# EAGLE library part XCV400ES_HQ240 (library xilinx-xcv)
xcv400es_hq240 edit this description Auto generated by make-symbol-device-package-bsdl.ulp Rev. 26 Source: xcv400es_hq240.bsd
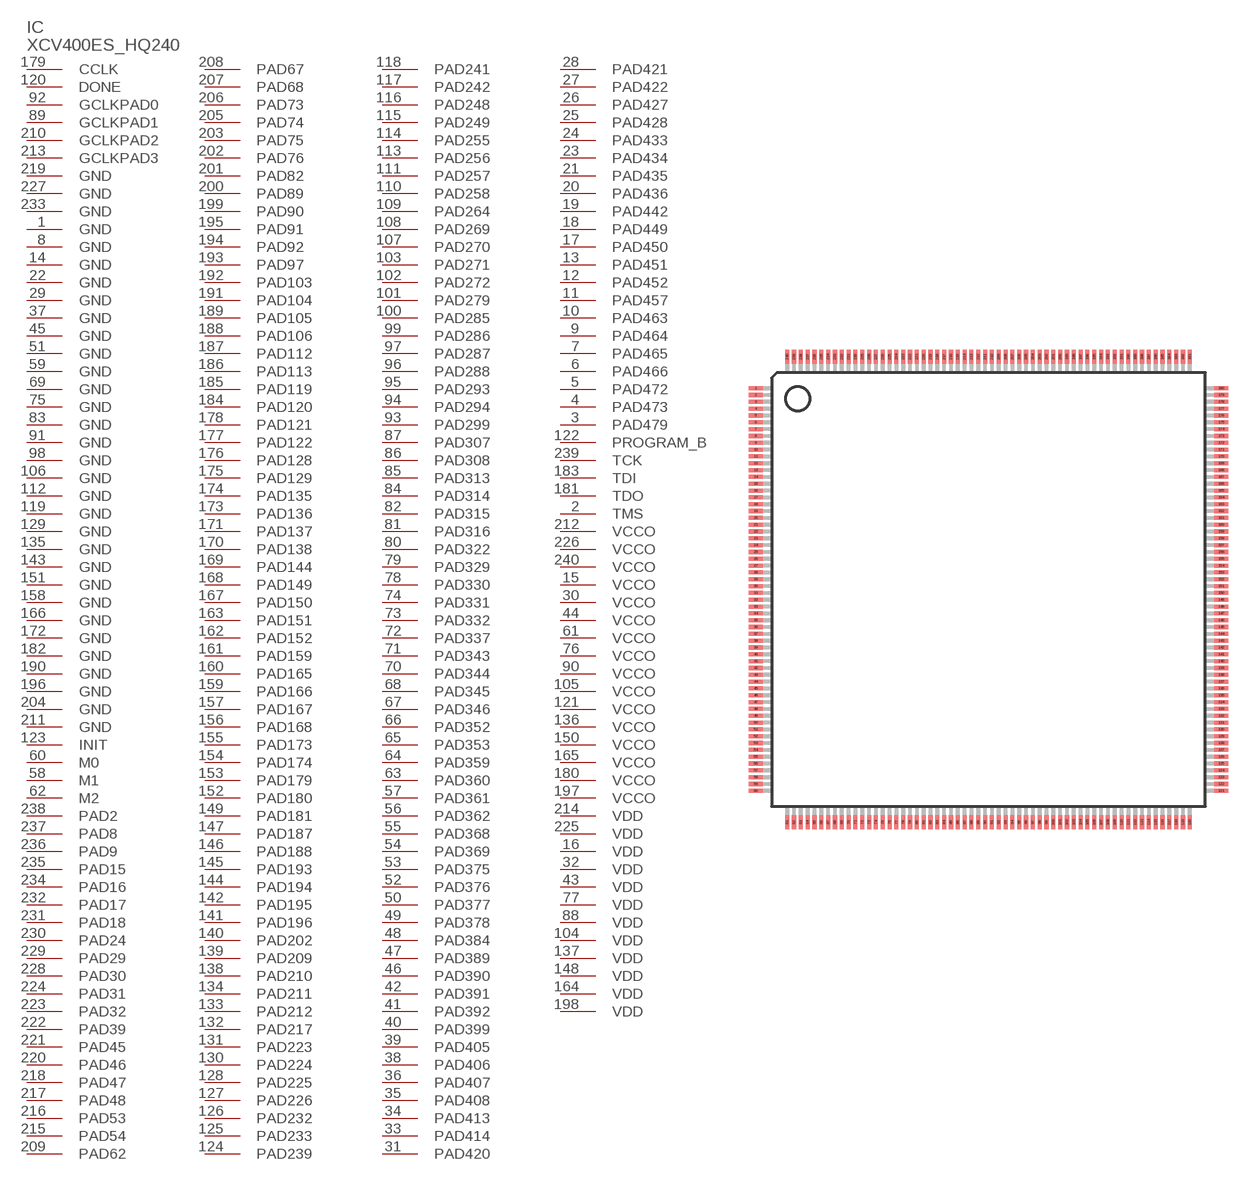
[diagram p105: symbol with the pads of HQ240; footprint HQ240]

Designator prefix IC

## XCV400ES_HQ240 (OC_FARNELL: unknown; OC_NEWARK: unknown)  [HQ240]
1  GND  pwr
2  TMS  in
3  PAD479
4  PAD473
5  PAD472
6  PAD466
7  PAD465
8  GND  pwr
9  PAD464
10  PAD463
11  PAD457
12  PAD452
13  PAD451
14  GND  pwr
15  VCCO  pwr
16  VDD  pwr
17  PAD450
18  PAD449
19  PAD442
20  PAD436
21  PAD435
22  GND  pwr
23  PAD434
24  PAD433
25  PAD428
26  PAD427
27  PAD422
28  PAD421
29  GND  pwr
30  VCCO  pwr
31  PAD420
32  VDD  pwr
33  PAD414
34  PAD413
35  PAD408
36  PAD407
37  GND  pwr
38  PAD406
39  PAD405
40  PAD399
41  PAD392
42  PAD391
43  VDD  pwr
44  VCCO  pwr
45  GND  pwr
46  PAD390
47  PAD389
48  PAD384
49  PAD378
50  PAD377
51  GND  pwr
52  PAD376
53  PAD375
54  PAD369
55  PAD368
56  PAD362
57  PAD361
58  M1  in
59  GND  pwr
60  M0  in
61  VCCO  pwr
62  M2  in
63  PAD360
64  PAD359
65  PAD353
66  PAD352
67  PAD346
68  PAD345
69  GND  pwr
70  PAD344
71  PAD343
72  PAD337
73  PAD332
74  PAD331
75  GND  pwr
76  VCCO  pwr
77  VDD  pwr
78  PAD330
79  PAD329
80  PAD322
81  PAD316
82  PAD315
83  GND  pwr
84  PAD314
85  PAD313
86  PAD308
87  PAD307
88  VDD  pwr
89  GCLKPAD1  in
90  VCCO  pwr
91  GND  pwr
92  GCLKPAD0  in
93  PAD299
94  PAD294
95  PAD293
96  PAD288
97  PAD287
98  GND  pwr
99  PAD286
100  PAD285
101  PAD279
102  PAD272
103  PAD271
104  VDD  pwr
105  VCCO  pwr
106  GND  pwr
107  PAD270
108  PAD269
109  PAD264
110  PAD258
111  PAD257
112  GND  pwr
113  PAD256
114  PAD255
115  PAD249
116  PAD248
117  PAD242
118  PAD241
119  GND  pwr
120  DONE
121  VCCO  pwr
122  PROGRAM_B  in
123  INIT
124  PAD239
125  PAD233
126  PAD232
127  PAD226
128  PAD225
129  GND  pwr
130  PAD224
131  PAD223
132  PAD217
133  PAD212
134  PAD211
135  GND  pwr
136  VCCO  pwr
137  VDD  pwr
138  PAD210
139  PAD209
140  PAD202
141  PAD196
142  PAD195
143  GND  pwr
144  PAD194
145  PAD193
146  PAD188
147  PAD187
148  VDD  pwr
149  PAD181
150  VCCO  pwr
151  GND  pwr
152  PAD180
153  PAD179
154  PAD174
155  PAD173
156  PAD168
157  PAD167
158  GND  pwr
159  PAD166
160  PAD165
161  PAD159
162  PAD152
163  PAD151
164  VDD  pwr
165  VCCO  pwr
166  GND  pwr
167  PAD150
168  PAD149
169  PAD144
170  PAD138
171  PAD137
172  GND  pwr
173  PAD136
174  PAD135
175  PAD129
176  PAD128
177  PAD122
178  PAD121
179  CCLK
180  VCCO  pwr
181  TDO  out
182  GND  pwr
183  TDI  in
184  PAD120
185  PAD119
186  PAD113
187  PAD112
188  PAD106
189  PAD105
190  GND  pwr
191  PAD104
192  PAD103
193  PAD97
194  PAD92
195  PAD91
196  GND  pwr
197  VCCO  pwr
198  VDD  pwr
199  PAD90
200  PAD89
201  PAD82
202  PAD76
203  PAD75
204  GND  pwr
205  PAD74
206  PAD73
207  PAD68
208  PAD67
209  PAD62
210  GCLKPAD2  in
211  GND  pwr
212  VCCO  pwr
213  GCLKPAD3  in
214  VDD  pwr
215  PAD54
216  PAD53
217  PAD48
218  PAD47
219  GND  pwr
220  PAD46
221  PAD45
222  PAD39
223  PAD32
224  PAD31
225  VDD  pwr
226  VCCO  pwr
227  GND  pwr
228  PAD30
229  PAD29
230  PAD24
231  PAD18
232  PAD17
233  GND  pwr
234  PAD16
235  PAD15
236  PAD9
237  PAD8
238  PAD2
239  TCK  in
240  VCCO  pwr

## Footprint HQ240 (pad centres in mm)
HQ240 Auto generated by make-symbol-device-package-bsdl.ulp Rev. 26
smd 1 x 0.3: 1 -17.05,14.75; 2 -17.05,14.25; 3 -17.05,13.75; 4 -17.05,13.25; 5 -17.05,12.75; 6 -17.05,12.25; 7 -17.05,11.75; 8 -17.05,11.25; 9 -17.05,10.75; 10 -17.05,10.25; 11 -17.05,9.75; 12 -17.05,9.25; 13 -17.05,8.75; 14 -17.05,8.25; 15 -17.05,7.75; 16 -17.05,7.25; 17 -17.05,6.75; 18 -17.05,6.25; 19 -17.05,5.75; 20 -17.05,5.25; 21 -17.05,4.75; 22 -17.05,4.25; 23 -17.05,3.75; 24 -17.05,3.25; 25 -17.05,2.75; 26 -17.05,2.25; 27 -17.05,1.75; 28 -17.05,1.25; 29 -17.05,0.75; 30 -17.05,0.25; 31 -17.05,-0.25; 32 -17.05,-0.75; 33 -17.05,-1.25; 34 -17.05,-1.75; 35 -17.05,-2.25; 36 -17.05,-2.75; 37 -17.05,-3.25; 38 -17.05,-3.75; 39 -17.05,-4.25; 40 -17.05,-4.75; 41 -17.05,-5.25; 42 -17.05,-5.75; 43 -17.05,-6.25; 44 -17.05,-6.75; 45 -17.05,-7.25; 46 -17.05,-7.75; 47 -17.05,-8.25; 48 -17.05,-8.75; 49 -17.05,-9.25; 50 -17.05,-9.75; 51 -17.05,-10.25; 52 -17.05,-10.75; 53 -17.05,-11.25; 54 -17.05,-11.75; 55 -17.05,-12.25; 56 -17.05,-12.75; 57 -17.05,-13.25; 58 -17.05,-13.75; 59 -17.05,-14.25; 60 -17.05,-14.75; 121 17.05,-14.75; 122 17.05,-14.25; 123 17.05,-13.75; 124 17.05,-13.25; 125 17.05,-12.75; 126 17.05,-12.25; 127 17.05,-11.75; 128 17.05,-11.25; 129 17.05,-10.75; 130 17.05,-10.25; 131 17.05,-9.75; 132 17.05,-9.25; 133 17.05,-8.75; 134 17.05,-8.25; 135 17.05,-7.75; 136 17.05,-7.25; 137 17.05,-6.75; 138 17.05,-6.25; 139 17.05,-5.75; 140 17.05,-5.25; 141 17.05,-4.75; 142 17.05,-4.25; 143 17.05,-3.75; 144 17.05,-3.25; 145 17.05,-2.75; 146 17.05,-2.25; 147 17.05,-1.75; 148 17.05,-1.25; 149 17.05,-0.75; 150 17.05,-0.25; 151 17.05,0.25; 152 17.05,0.75; 153 17.05,1.25; 154 17.05,1.75; 155 17.05,2.25; 156 17.05,2.75; 157 17.05,3.25; 158 17.05,3.75; 159 17.05,4.25; 160 17.05,4.75; 161 17.05,5.25; 162 17.05,5.75; 163 17.05,6.25; 164 17.05,6.75; 165 17.05,7.25; 166 17.05,7.75; 167 17.05,8.25; 168 17.05,8.75; 169 17.05,9.25; 170 17.05,9.75; 171 17.05,10.25; 172 17.05,10.75; 173 17.05,11.25; 174 17.05,11.75; 175 17.05,12.25; 176 17.05,12.75; 177 17.05,13.25; 178 17.05,13.75; 179 17.05,14.25; 180 17.05,14.75
smd 0.3 x 1: 61 -14.75,-17.05; 62 -14.25,-17.05; 63 -13.75,-17.05; 64 -13.25,-17.05; 65 -12.75,-17.05; 66 -12.25,-17.05; 67 -11.75,-17.05; 68 -11.25,-17.05; 69 -10.75,-17.05; 70 -10.25,-17.05; 71 -9.75,-17.05; 72 -9.25,-17.05; 73 -8.75,-17.05; 74 -8.25,-17.05; 75 -7.75,-17.05; 76 -7.25,-17.05; 77 -6.75,-17.05; 78 -6.25,-17.05; 79 -5.75,-17.05; 80 -5.25,-17.05; 81 -4.75,-17.05; 82 -4.25,-17.05; 83 -3.75,-17.05; 84 -3.25,-17.05; 85 -2.75,-17.05; 86 -2.25,-17.05; 87 -1.75,-17.05; 88 -1.25,-17.05; 89 -0.75,-17.05; 90 -0.25,-17.05; 91 0.25,-17.05; 92 0.75,-17.05; 93 1.25,-17.05; 94 1.75,-17.05; 95 2.25,-17.05; 96 2.75,-17.05; 97 3.25,-17.05; 98 3.75,-17.05; 99 4.25,-17.05; 100 4.75,-17.05; 101 5.25,-17.05; 102 5.75,-17.05; 103 6.25,-17.05; 104 6.75,-17.05; 105 7.25,-17.05; 106 7.75,-17.05; 107 8.25,-17.05; 108 8.75,-17.05; 109 9.25,-17.05; 110 9.75,-17.05; 111 10.25,-17.05; 112 10.75,-17.05; 113 11.25,-17.05; 114 11.75,-17.05; 115 12.25,-17.05; 116 12.75,-17.05; 117 13.25,-17.05; 118 13.75,-17.05; 119 14.25,-17.05; 120 14.75,-17.05; 181 14.75,17.05; 182 14.25,17.05; 183 13.75,17.05; 184 13.25,17.05; 185 12.75,17.05; 186 12.25,17.05; 187 11.75,17.05; 188 11.25,17.05; 189 10.75,17.05; 190 10.25,17.05; 191 9.75,17.05; 192 9.25,17.05; 193 8.75,17.05; 194 8.25,17.05; 195 7.75,17.05; 196 7.25,17.05; 197 6.75,17.05; 198 6.25,17.05; 199 5.75,17.05; 200 5.25,17.05; 201 4.75,17.05; 202 4.25,17.05; 203 3.75,17.05; 204 3.25,17.05; 205 2.75,17.05; 206 2.25,17.05; 207 1.75,17.05; 208 1.25,17.05; 209 0.75,17.05; 210 0.25,17.05; 211 -0.25,17.05; 212 -0.75,17.05; 213 -1.25,17.05; 214 -1.75,17.05; 215 -2.25,17.05; 216 -2.75,17.05; 217 -3.25,17.05; 218 -3.75,17.05; 219 -4.25,17.05; 220 -4.75,17.05; 221 -5.25,17.05; 222 -5.75,17.05; 223 -6.25,17.05; 224 -6.75,17.05; 225 -7.25,17.05; 226 -7.75,17.05; 227 -8.25,17.05; 228 -8.75,17.05; 229 -9.25,17.05; 230 -9.75,17.05; 231 -10.25,17.05; 232 -10.75,17.05; 233 -11.25,17.05; 234 -11.75,17.05; 235 -12.25,17.05; 236 -12.75,17.05; 237 -13.25,17.05; 238 -13.75,17.05; 239 -14.25,17.05; 240 -14.75,17.05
